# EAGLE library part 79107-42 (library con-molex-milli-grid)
RECEPTACAL
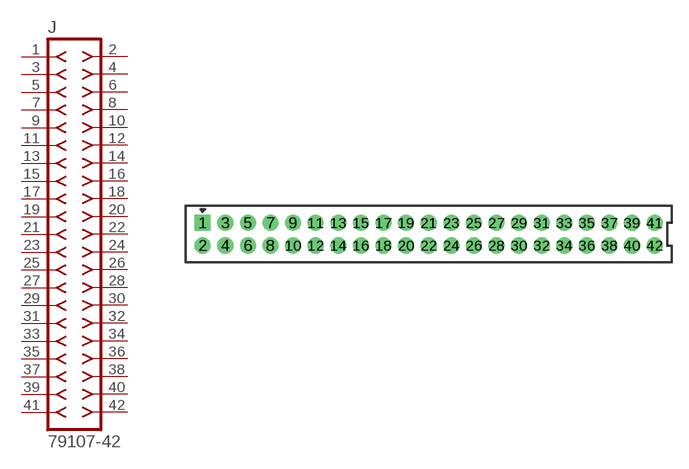
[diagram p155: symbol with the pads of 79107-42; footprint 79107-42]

Designator prefix J

## 79107-42  [79107-42]
1  1  pas
2  2  pas
3  3  pas
4  4  pas
5  5  pas
6  6  pas
7  7  pas
8  8  pas
9  9  pas
10  10  pas
11  11  pas
12  12  pas
13  13  pas
14  14  pas
15  15  pas
16  16  pas
17  17  pas
18  18  pas
19  19  pas
20  20  pas
21  21  pas
22  22  pas
23  23  pas
24  24  pas
25  25  pas
26  26  pas
27  27  pas
28  28  pas
29  29  pas
30  30  pas
31  31  pas
32  32  pas
33  33  pas
34  34  pas
35  35  pas
36  36  pas
37  37  pas
38  38  pas
39  39  pas
40  40  pas
41  41  pas
42  42  pas

## Footprint 79107-42 (pad centres in mm)
RECEPTACAL Dual Row, Vertical, Through-Hole
drill 0.914 square: 1 -20,1
drill 0.914: 2 -20,-1; 3 -18,1; 4 -18,-1; 5 -16,1; 6 -16,-1; 7 -14,1; 8 -14,-1; 9 -12,1; 10 -12,-1; 11 -10,1; 12 -10,-1; 13 -8,1; 14 -8,-1; 15 -6,1; 16 -6,-1; 17 -4,1; 18 -4,-1; 19 -2,1; 20 -2,-1; 21 0,1; 22 0,-1; 23 2,1; 24 2,-1; 25 4,1; 26 4,-1; 27 6,1; 28 6,-1; 29 8,1; 30 8,-1; 31 10,1; 32 10,-1; 33 12,1; 34 12,-1; 35 14,1; 36 14,-1; 37 16,1; 38 16,-1; 39 18,1; 40 18,-1; 41 20,1; 42 20,-1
